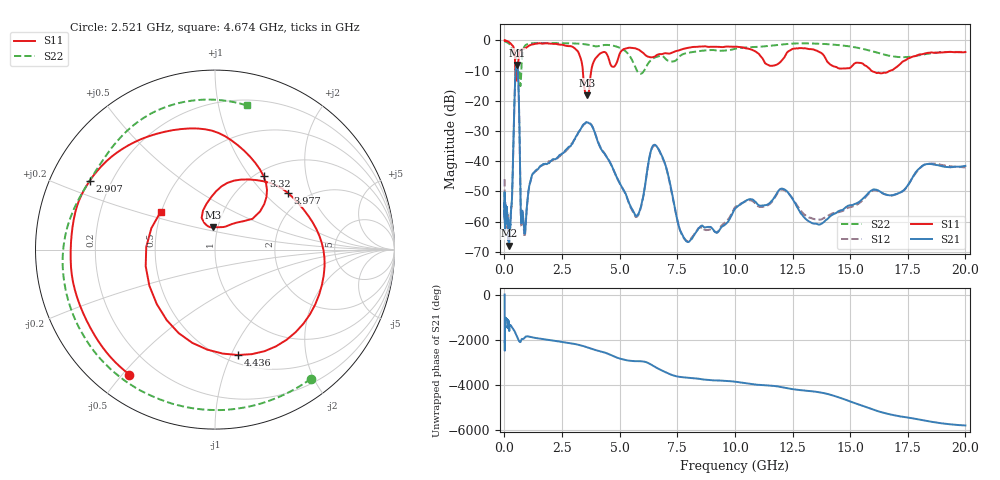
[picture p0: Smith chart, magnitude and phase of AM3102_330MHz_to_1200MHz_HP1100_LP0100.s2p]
! Date/Time: Tue, Sep 11, 2018 5:21 PM
! Network Analyzer: Agilent Technologies E8362B Rev: A.07.50.63
! Sweep from 0.010 to 20.000 GHz, 1601 Points, Sweep Type: LOG
! Power Supply: 4.949 V, 0.001 A
# Hz S DB R 50
!freq MagS11 AngS11 MagS21 AngS21 MagS12 AngS12 MagS22 AngS22
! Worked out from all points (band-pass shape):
!   1601 points, 10 MHz to 20 GHz, reference 50 ohm
!   highest |S21| = -8.15 dB at 546 MHz (marker M1); lowest = -67.9 dB at 196.6 MHz (marker M2)
!   |S21| within 3 dB of the highest: 478.5 MHz to 593.6 MHz (115.1 MHz wide, 21.5 % of centre)
!   lowest |S11| = -18.1 dB at 3.599 GHz (marker M3), VSWR 1.28, Z = 47.6 + j12 ohm
!   |S11| at or under -10 dB: 472.4 MHz to 523.4 MHz (51 MHz wide, 10.2 % of centre); 3.403 GHz to 3.769 GHz (366.3 MHz wide, 10.2 % of centre); 15.92 GHz to 16.76 GHz (844.9 MHz wide, 5.17 % of centre)
!   |S22| runs from -15.1 to -0.2 dB; largest |S21 - S12| = 0.0059
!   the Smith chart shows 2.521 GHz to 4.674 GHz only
!   S11 on the Smith chart (normalised r, x): 2.521 GHz: 0.11, -0.52; 2.907 GHz: 0.12, +0.25; 3.32 GHz: 1.09, +1.17; 3.977 GHz: 1.63, +1.40; 4.436 GHz: 0.58, -1.06; 4.674 GHz: 0.50, +0.24
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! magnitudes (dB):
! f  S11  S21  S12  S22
! 10 MHz  0.0  -59.1  -46.0  -0.2
! 35.55 MHz  -0.1  -59.4  -60.5  -0.3
! 126.4 MHz  -0.3  -58.9  -57.9  -0.7
! 196.6 MHz  -0.6  -67.9  -68.1  -1.1
! 328.4 MHz  -1.6  -52.6  -52.8  -3.1
! 447.2 MHz  -4.5  -17.7  -17.7  -4.3
! 546 MHz  -9.1  -8.1  -8.2  -9.1
! 620.7 MHz  -5.3  -17.2  -17.2  -10.5
! 736.5 MHz  -3.0  -60.5  -61.6  -9.5
! 886.4 MHz  -2.7  -63.9  -64.7  -1.9
! 1.59 GHz  -1.0  -41.5  -41.4  -0.9
! 2.521 GHz  -1.5  -37.3  -37.4  -1.0
! 2.907 GHz  -2.0  -34.5  -34.3  -1.0
! 3.32 GHz  -6.2  -29.2  -29.2  -1.1
! 3.599 GHz  -18.1  -27.2  -27.0  -1.4
! 3.977 GHz  -5.8  -31.8  -31.7  -2.0
! 4.436 GHz  -4.4  -38.6  -38.5  -1.5
! 4.674 GHz  -8.7  -41.8  -41.9  -1.7
! 5.652 GHz  -2.6  -57.5  -57.8  -8.4
! 6.549 GHz  -5.2  -34.6  -34.8  -5.6
! 7.958 GHz  -2.5  -66.7  -66.6  -4.1
! 20 GHz  -3.9  -41.5  -42.0  -3.8
